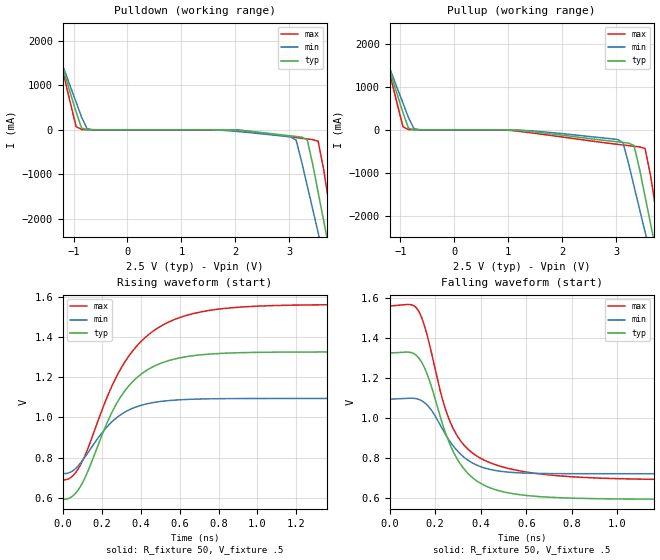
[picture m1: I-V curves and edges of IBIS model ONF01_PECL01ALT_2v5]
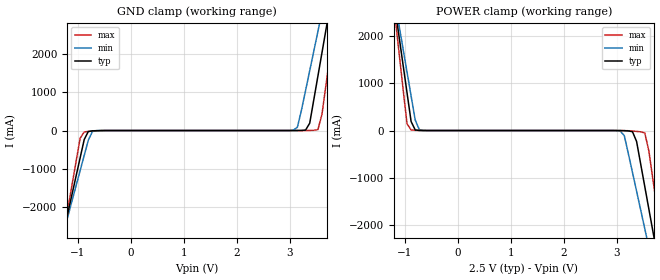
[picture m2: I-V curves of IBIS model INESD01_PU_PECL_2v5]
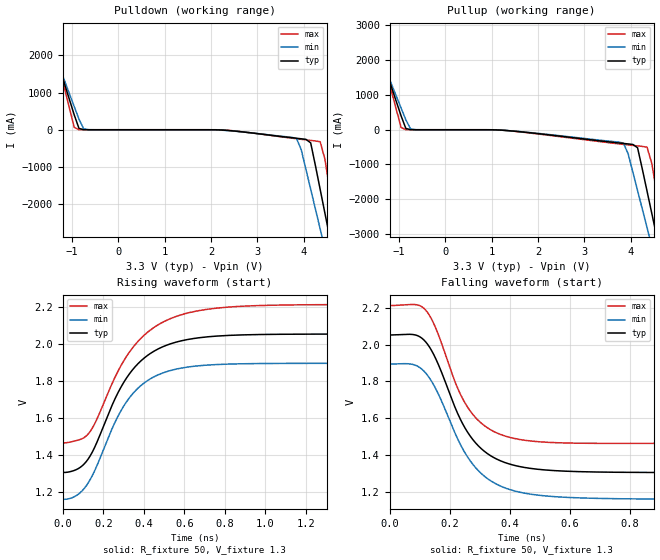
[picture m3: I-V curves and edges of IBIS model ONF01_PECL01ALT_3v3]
|   This file is an IBIS representation of the   |
|   Integrated Devices Technology, Inc.   |
|   ICS85320I   |
|   LVCMOS/LVTTL-TO-DIFFERENTIAL 3.3V, 2.5V LVPECL TRANSLATOR   |
[IBIS Ver]   4.1
[File name]   85320i.ibs
[File Rev]   1.0
[Date]   30 Dec 2008 | Last modified
[Source]   Originated at Integrated Devices Technology, Inc.
[Disclaimer]
IDT hereby grants the user of this IBIS model a non-exclusive,
nontransferable license to use this IBIS model under the following terms.
Before using this IBIS model, the user should read this license.
If the user does not accept these terms,  the IBIS model should be
returned to IDT within 30 days.
   The user is granted this license only to use the IBIS model and
is not granted rights to sell, load, rent, lease or license the IBIS
model in whole or in part, or in modified form to anyone other than
user. User may modify the IBIS model to suit its specific
applications but rights to derivative works and such modifications
shall belong to IDT.
   This IBIS model is provided on an "AS IS" basis and IDT makes
absolutely no warranty with respect to the information contained
herein. IDT DISCLAIMS AND CUSTOMER WAIVES ALL WARRANTIES, EXPRESS
OR IMPLIED, INCLUDING WARRANTIES OF MERCHANTABILITY OR FITNESS FOR
A PARTICULAR PURPOSE. The entire risk as to quality and performance
is with the Customer. ACCORDINGLY, IN NO EVENT SHALL THE COMPANY BE
LIABLE FOR ANY DAMAGES, WHETHER IN CONTRACT OR TORT,INCLUDING ANY
LOST PROFITS OR OTHER INCIDENTAL, CONSEQUENTIAL, EXEMPLARY, OR
PUNITIVE DAMAGES ARISING OUT OF THE USE OR APPLICATION OF THE IBIS
model provided in this package. Further, IDT reserves the right to
make changes without notice to any product herein to improve
reliability, function, or design. IDT does not convey any license
under patent rights or any other intellectual property rights,
including those of third parties.
   IDT is not obligated to provide maintenance or support
for the licensed IBIS model.
[Copyright]   Copyright 2003 by Integrated Devices Technology, Inc.
[Component]   ICS85320I
[Manufacturer] Integrated Devices Technology, Inc.
[Package]
|SOIC 8 Lead
|   typ   min   max
R_pkg   57.05m   55.5m   58.6m
L_pkg   1.769nH   1.570nH   1.968nH
C_pkg   0.269pF   0.252pF   0.286pF
[Pin]   signal_name   model_name   R_pin   L_pin   C_pin
1   NC   NC   58.6m   1.968n   0.286p
2   Q   ONF01_PECL01ALT   55.5m   1.570n   0.252p
3   nQ   ONF01_PECL01ALT   55.5m   1.570n   0.252p
4   NC   NC   56.6m   1.968n   0.286p
5   VEE   GND   58.6m   1.968n   0.286p
6   NC   NC   55.5m   1.570n   0.252p
7   CLK   INESD01_PU_PECL   55.5m   1.570n   0.252p
8   VCC   POWER   56.6m   1.968n   0.286p
[Diff Pin]  inv_pin  vdiff tdelay_typ tdelay_min  tdelay_max
2   3   NA   0  0  0
[Model Selector] ONF01_PECL01ALT
ONF01_PECL01ALT_2v5  Buffer selection for 2v5
ONF01_PECL01ALT_3v3  Buffer selection for 3v3
[Model Selector] INESD01_PU_PECL
INESD01_PU_PECL_2v5  Buffer selection for 2v5
INESD01_PU_PECL_3v3  Buffer selection for 3v3
| Models and submodels in the file (4): ONF01_PECL01ALT_2v5 (Output_ECL), INESD01_PU_PECL_2v5 (Input), ONF01_PECL01ALT_3v3 (Output_ECL), INESD01_PU_PECL_3v3 (Input)
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[Model] ONF01_PECL01ALT_2v5
Model_type  Output_ECL
Polarity   Non-Inverting
Vmeas = .975
Rref = 50
Cref = 0
Vref = .5
|Variable  typ   min   max
C_comp   2p   1.5p   2.5p
[Voltage Range]   2.5   2.375   2.625
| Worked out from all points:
|   rising waveform, R_fixture 50, V_fixture .5: 20-80 % time 228ps typ, 199ps min, 276ps max; typ from 0.592 V to 1.33 V
|   falling waveform, R_fixture 50, V_fixture .5: 20-80 % time 153ps typ, 140ps min, 156ps max; typ from 1.33 V to 0.592 V
| Open source, no load
|  Voltage   I(typ)   I(min)   I(max)
[Pullup]
-3.3V     9.786A     8.425A     12.06A
-1.463V   2.432A     2.308A     2.661A
-952.6mV  398mA      618.5mA    68.87mA
-850.5mV  36.63mA    281.6mA    4.032mA
-646.4mV  229.3uA    964.8uA    177.5uA
3.028V    -282.4mA   -226.8mA   -340.1mA
3.13V     -296.5mA   -301.7mA   -355.4mA
3.334V    -367.3mA   -1.316A    -385.1mA
3.538V    -1.551A    -2.377A    -435.3mA
3.64V     -2.187A    -2.908A    -1.066A
3.844V    -3.46A     -3.969A    -2.688A
6.6V      -20.66A    -18.32A    -24.61A
[Pulldown]
-3.3V     9.786A     8.425A     12.06A
-1.463V   2.432A     2.308A     2.661A
-1.361V   2.024A     1.97A      2.139A
-952.6mV  398mA      618.5mA    68.87mA
-850.5mV  36.63mA    281.6mA    4.032mA
3.028V    -137.6mA   -160.7mA   -160.7mA
3.13V     -151.4mA   -235.1mA   -176.3mA
3.334V    -221.9mA   -1.249A    -206.7mA
3.538V    -1.406A    -2.31A     -257.4mA
3.64V     -2.042A    -2.84A     -888.8mA
3.844V    -3.314A    -3.9A      -2.51A
6.6V      -20.58A    -18.26A    -24.54A
[Ramp]
|   typ   min   max
dV/dt_r   0.586/0.368n   0.299/0.313n   0.698/0.446n
dV/dt_f   0.586/0.258n   0.299/0.226n   0.698/0.290n
R_load =   50.0000
[Rising Waveform]
R_fixture = 50
V_fixture = .5   | VCC_typ - 2V
V_fixture_max = 0.625   | VCC_max - 2V
V_fixture_min = 0.375   | VCC_min - 2V
C_fixture = 0.0p
| Time   typ   min   max
0s        592.5mV    720.8mV    689.3mV
46.2ps    605.5mV    731.1mV    704.8mV
92.4ps    659.4mV    774.5mV    766.4mV
241.5ps   1.003V     967.6mV    1.133V
323.4ps   1.138V     1.029V     1.283V
426.3ps   1.231V     1.066V     1.4V
552.3ps   1.285V     1.084V     1.478V
711.9ps   1.312V     1.092V     1.525V
940.8ps   1.323V     1.094V     1.551V
1.999ns   1.326V     1.094V     1.562V
[Falling Waveform]
R_fixture = 50
V_fixture = .5   | VCC_typ - 2V
V_fixture_max = 0.625   | VCC_max - 2V
V_fixture_min = 0.375   | VCC_min - 2V
C_fixture = 0.0p
0s        1.326V     1.094V     1.562V
92.4ps    1.328V     1.099V     1.568V
123.9ps   1.306V     1.095V     1.541V
168ps     1.209V     1.061V     1.4V
231ps     973.8mV    945.4mV    1.097V
277.2ps   835.9mV    862.7mV    951mV
348.6ps   716.5mV    784.8mV    838.7mV
447.3ps   647.2mV    740.6mV    773mV
865.2ps   596.5mV    720.8mV    701.4mV
1.999ns   592.4mV    720.7mV    689.3mV
[Model] INESD01_PU_PECL_2v5
Model_type  Input
Polarity   Non-Inverting
Vinl = 0.9
Vinh = 1.6V
|   typ   min   max
C_comp   2pF   1.5pF   2.5pF
|   typ   min   max
[Voltage range]  2.5V   2.375V   2.625V
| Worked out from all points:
|   GND clamp passes 1 mA (typ) near -0.54 V on its own axis
|   POWER clamp passes 1 mA (typ) near -0.67 V on its own axis
[GND_clamp]
|Voltage   I(typ)   I(min)   I(max)
-2.5V     -10.33A    -9.044A    -12.47A
-1.263V   -2.632A    -2.639A    -2.655A
-953.6mV  -711.7mA   -1.044A    -200.4mA
-876.3mV  -232.8mA   -646mA     -36.9mA
-644.3mV  -3.744mA   -3.442mA   -8.163mA
3.067V    100.7uA    7.657mA    8.292uA
3.144V    453.6uA    86.78mA    24.43uA
3.376V    191.1mA    1.558A     2.391mA
3.531V    1.418A     2.581A     23.29mA
3.686V    2.649A     3.605A     1.215A
3.84V     3.882A     4.631A     2.791A
5V        13.16A     12.34A     14.65A
[POWER_clamp]
|Voltage   I(typ)   I(min)   I(max)
-2.5V     13.16A     11.51A     15.93A
-1.186V   2.649A     2.777A     2.489A
-1.108V   2.034A     2.265A     1.701A
-953.6mV  804mA      1.243A     144.3mA
-876.3mV  191.1mA    733mA      11.81mA
-644.3mV  453.6uA    1.831mA    349.6uA
3.067V    -1.275mA   -11.3mA    -266.4uA
3.299V    -24.55mA   -891.1mA   -10.77mA
3.531V    -1.191A    -2.086A    -51.94mA
3.686V    -2.151A    -2.885A    -1.049A
3.84V     -3.112A    -3.684A    -2.276A
5V        -10.33A    -9.692A    -11.48A
[Model] ONF01_PECL01ALT_3v3
Model_type  Output_ECL
Polarity   Non-Inverting
Vmeas = 1.636
Rref = 50
Cref = 0
Vref = 1.3
|Variable  typ   min   max
C_comp   2p   1.5p   2.5p
[Voltage Range]   3.3   3.135   3.465
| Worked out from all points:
|   rising waveform, R_fixture 50, V_fixture 1.3: 20-80 % time 218ps typ, 206ps min, 242ps max; typ from 1.31 V to 2.05 V
|   falling waveform, R_fixture 50, V_fixture 1.3: 20-80 % time 134ps typ, 143ps min, 120ps max; typ from 2.05 V to 1.31 V
| Open source, no load
|  Voltage   I(typ)   I(min)   I(max)
[Pullup]
-3.3V     9.786A     8.45A      12.03A
-1.667V   3.247A     2.997A     3.691A
-1.565V   2.839A     2.657A     3.17A
-952.6mV  398mA      622.1mA    64.71mA
-850.5mV  36.63mA    284.2mA    1.532mA
-646.4mV  229.3uA    1.611mA    19.07uA
3.844V    -394.4mA   -383.6mA   -421.3mA
4.151V    -517.8mA   -1.749A    -465.4mA
4.355V    -1.764A    -2.812A    -500.3mA
4.559V    -3.036A    -3.875A    -1.773A
4.763V    -4.308A    -4.937A    -3.393A
6.6V      -15.79A    -14.52A    -18.03A
[Pulldown]
-3.3V     9.786A     8.45A      12.03A
-1.565V   2.839A     2.657A     3.17A
-1.463V   2.432A     2.317A     2.65A
-952.6mV  398mA      622.1mA    64.71mA
-850.5mV  36.63mA    284.2mA    1.532mA
-646.4mV  229.3uA    1.611mA    19.07uA
3.844V    -229.1mA   -232.1mA   -241.8mA
4.151V    -352.7mA   -1.598A    -286.7mA
4.355V    -1.599A    -2.66A     -322.1mA
4.559V    -2.871A    -3.722A    -1.595A
4.763V    -4.144A    -4.785A    -3.217A
6.6V      -15.69A    -14.41A    -17.97A
[Ramp]
|   typ   min   max
dV/dt_r   0.45V/0.37ns   0.45V/0.405ns   0.45V/0.27ns
dV/dt_f   0.45V/0.37ns   0.45V/0.405ns   0.45V/0.27ns
R_load =   50.0000
[Rising Waveform]
R_fixture = 50
V_fixture = 1.3   | VCC_typ - 2V
V_fixture_max = 1.465   | VCC_max - 2V
V_fixture_min = 1.135   | VCC_min - 2V
C_fixture = 0.0p
| Time   typ   min   max
0s        1.306V     1.161V     1.465V
70ps      1.323V     1.183V     1.479V
128ps     1.383V     1.254V     1.517V
258ps     1.703V     1.577V     1.819V
316ps     1.817V     1.689V     1.934V
398ps     1.919V     1.785V     2.042V
504ps     1.988V     1.846V     2.121V
658ps     2.03V      1.879V     2.175V
875ps     2.047V     1.891V     2.201V
2ns       2.052V     1.894V     2.211V
[Falling Waveform]
R_fixture = 50
V_fixture = 1.3   | VCC_typ - 2V
V_fixture_max = 1.465   | VCC_max - 2V
V_fixture_min = 1.135   | VCC_min - 2V
C_fixture = 0.0p
0s        2.052V     1.894V     2.211V
76ps      2.055V     1.893V     2.217V
118ps     2.018V     1.85V      2.19V
150ps     1.936V     1.772V     2.103V
222ps     1.644V     1.505V     1.782V
264ps     1.514V     1.38V      1.65V
326ps     1.409V     1.274V     1.549V
410ps     1.348V     1.21V      1.493V
708ps     1.309V     1.166V     1.465V
2ns       1.306V     1.161V     1.465V
